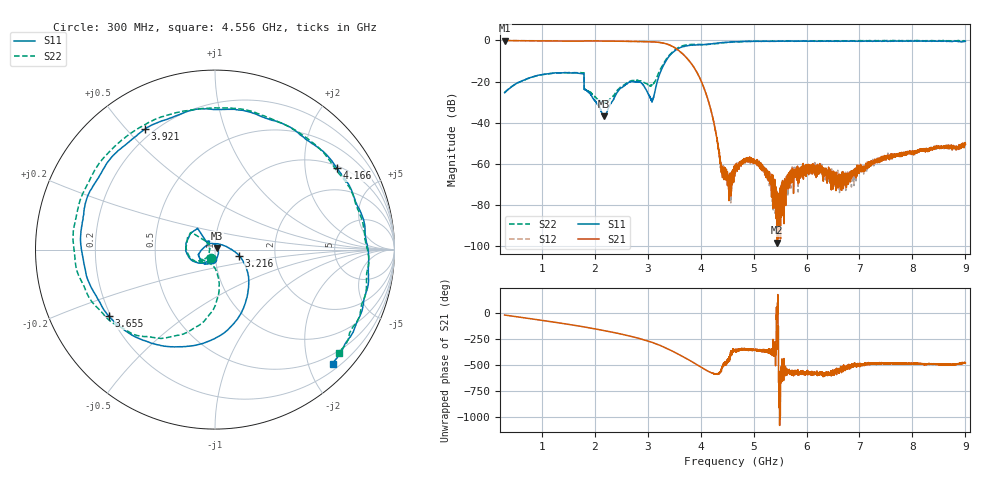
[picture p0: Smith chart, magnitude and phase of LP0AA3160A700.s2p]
!Agilent Technologies,E8358A,US41080443,A.07.50.56
!Agilent E8358A: A.07.50.56
!Date: Monday, December 14, 2015 10:37:38
!Correction: S11(Full 2 Port(1,2))
!S21(Full 2 Port(1,2))
!S12(Full 2 Port(1,2))
!S22(Full 2 Port(1,2))
!S2P File: Measurements: S11, S21, S12, S22:
# Hz S  dB  R 50
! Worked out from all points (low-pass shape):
!   6401 points, 300 MHz to 9 GHz, reference 50 ohm
!   highest |S21| = -0.07 dB at 302.7 MHz (marker M1); lowest = -98.4 dB at 5.449 GHz (marker M2)
!   |S21| within 3 dB of the highest: start of sweep to 3.479 GHz
!   lowest |S11| = -36.9 dB at 2.179 GHz (marker M3), VSWR 1.03, Z = 51.3 + j0.66 ohm
!   |S11| at or under -10 dB: start of sweep to 3.346 GHz
!   |S22| runs from -30.7 to 0.0 dB; largest |S21 - S12| = 0.014
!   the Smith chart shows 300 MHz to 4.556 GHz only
!   S11 on the Smith chart (normalised r, x): 300 MHz: 0.96, -0.10; 3.216 GHz: 1.31, -0.09; 3.655 GHz: 0.19, -0.28; 3.921 GHz: 0.17, +0.56; 4.166 GHz: 1.08, +2.93; 4.556 GHz: 0.32, -2.42
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3e8  -25.39 -110.2  -0.07 -21.5  -0.06 -21.4  -25.43 -112.8
3.027188e8  -25.36 -110.2  -0.07 -21.8  -0.07 -21.6  -25.36 -113.1
1.072125e9  -16.38 -164.2  -0.26 -77.5  -0.24 -77.2  -16.44 -169.3
1.750453e9  -16.13 136.2  -0.35 -130.6  -0.32 -130.2  -15.71 145.9
2.178656e9  -36.86 26.6  -0.31 -170.0  -0.29 -169.6  -30.61 -179.4
2.676188e9  -20.03 -126.8  -0.49 135.8  -0.48 136.3  -19.74 -141.8
3.077203e9  -29.45 93.2  -0.70 78.6  -0.69 79.1  -21.61 -111.7
3.200906e9  -18.31 -9.0  -0.91 55.4  -0.89 56.1  -16.22 -83.5
3.215859e9  -17.16 -13.8  -0.97 52.5  -0.95 53.1  -15.35 -82.7
3.421125e9  -7.26 -77.4  -2.34 5.3  -2.31 5.9  -6.89 -105.0
3.654938e9  -3.11 -148.0  -6.35 -55.9  -6.33 -55.1  -2.71 -153.9
3.921375e9  -2.21 120.3  -15.07 -133.0  -15.05 -132.4  -1.92 134.5
4.166062e9  -1.77 33.8  -31.17 155.4  -31.10 155.6  -1.90 51.3
4.401234e9  -1.08 -20.9  -60.99 -174.0  -61.51 -177.2  -1.25 -12.7
4.556203e9  -0.79 -44.2  -70.74 -60.2  -70.74 -87.8  -0.93 -40.0
4.65e9  -0.69 -55.2  -64.21 5.3  -64.38 3.9  -0.74 -52.6
5.10675e9  -0.44 -92.4  -59.57 3.0  -60.74 -0.6  -0.44 -89.1
5.449312e9  -0.35 -112.6  -98.35 35.2  -76.30 -54.2  -0.31 -108.6
6.100453e9  -0.39 -145.5  -63.42 161.4  -63.59 133.3  -0.36 -144.6
6.651e9  -0.39 -168.5  -66.87 -177.9  -66.15 -161.5  -0.27 -169.5
7.550906e9  -0.38 169.5  -56.04 -123.4  -56.40 -121.3  -0.15 168.1
9e9  -0.40 150.5  -50.55 -118.2  -50.36 -114.8  -0.26 137.0
